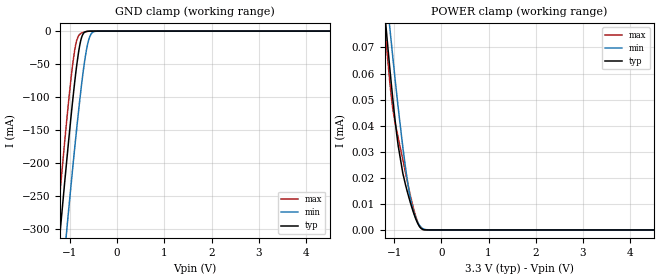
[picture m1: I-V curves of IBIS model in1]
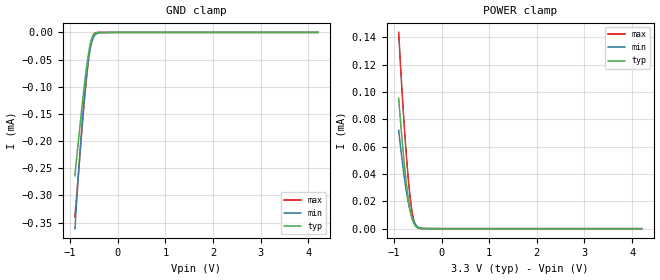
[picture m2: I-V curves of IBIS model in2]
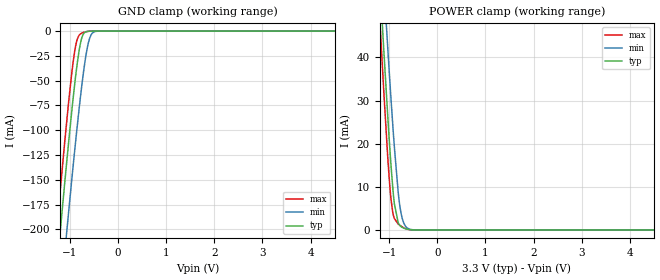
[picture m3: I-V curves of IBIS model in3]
|Texas Instruments Incorporated
|TPS53688 Dual-Channel (8+0, 7+1, 6+2, 5+3, 4+4 Phsases) D-CAP+ tm , Step Down
|Digital Multiphase Controller with VR13.HC and SVID
[IBIS Ver]   4.1
[File name]   tps53688.ibs
[Date]   25/04/2019
[File Rev]   1.0
[Source]
| Texas Instruments Incorporated.
| Analog-eLab Design Center, HPA
| 12500 TI Blvd
| Dallas, TX -75243
[Notes]   Revision History:
| Rev 1.0: 25/04/2019
| - Initial version of the model
| - Model generated from simulations in SPECTRE
| - C_comp although listed in numerical order of value are
|   obtained from varying PVT conditions. For PVT conditions for
|   each specific value refer the buffer description under
|   respective [Model]. IBIS model user is responsible for using
|   appropriate C_comp to simulate for Signal Integrity.
[Disclaimer]
| This model is designed as an aid for customers of Texas Instruments.
| TI and its licensors and suppliers make no warranties, either expressed
| or implied, with respect to this  model, including the warranties of
| merchantability or fitness for a particular purpose. The model is
| provided solely on an "as is" basis. The entire risk as to its quality
| and performance is with the customer.
| This model is subject to change without notice. Texas Instruments
| Incorporated is not responsible for updating this model.
[Copyright]
(C) Copyright 2019 Texas Instruments Incorporated.All rights reserved.
|  Component TPS53688RSB 40-Pin WQFN -RSB package
|  Part # TPS53688RSB
[Component]   TPS53688RSB
[Manufacturer]   TI
[Package]   |40 WQFN -RSB package
|   typ   min   max
R_pkg   0.05   0.04   0.06
L_pkg   1.0nH   0.8nH   1.2nH
C_pkg   0.2pF   0.16pF   0.24pF
[Pin] signal_name   model_name   R_pin   L_pin   C_pin
1   APWM8/BPWM1   out   NA   NA   NA
2   APWM7/BPWM2   out   NA   NA   NA
3   APWM6/BPWM3   out   NA   NA   NA
4   APWM5/BPWM4   out   NA   NA   NA
5   APWM4   out   NA   NA   NA
6   APWM3   out   NA   NA   NA
7   APWM2   out   NA   NA   NA
8   APWM1   out   NA   NA   NA
9   SMB_DIO   iood1   NA   NA   NA
10   SMB_CLK   iood1   NA   NA   NA
11   SMB_ALERTB   od1   NA   NA   NA
12   AVR_RDY   od2   NA   NA   NA
13   AVR_EN   in1   NA   NA   NA
14   VR_HOTB   od3   NA   NA   NA
15   PIN_ALT/PSYS_CRITB   od4   NA   NA   NA
16   BVR_RDY   od2   NA   NA   NA
17   SV_CLK   in2   NA   NA   NA
18   SV_DIO   iood2   NA   NA   NA
19   SV_ALERTB   iood2   NA   NA   NA
20   BVR_EN/VCCIO   in3   NA   NA   NA
21   AVSP   NC   NA   NA   NA
22   AVSN   NC   NA   NA   NA
23   ACSP1   NC   NA   NA   NA
24   ACSP2   NC   NA   NA   NA
25   ACSP3   NC   NA   NA   NA
26   ACSP4   NC   NA   NA   NA
27   ACSP5/BCSP4   NC   NA   NA   NA
28   ACSP6/BCSP3   NC   NA   NA   NA
29   ACSP7/BCSP2   NC   NA   NA   NA
30   ACSP8/BCSP1   NC   NA   NA   NA
31   BVSN   NC   NA   NA   NA
32   BVSP   NC   NA   NA   NA
33   VR_FAULTB   od5   NA   NA   NA
34   ADDR_CONFIG   NC   NA   NA   NA
35   BTSEN/TSEN   NC   NA   NA   NA
36   ATSEN/ISYS_IN   NC   NA   NA   NA
37   CSPIN   NC   NA   NA   NA
38   VIN_CSNIN   NC   NA   NA   NA
39   VCC   POWER   NA   NA   NA
40   VREF   NC   NA   NA   NA
| Models and submodels in the file (11): in1 (Input), in2 (Input), in3 (Input), iood1 (I/O_open_drain), iood2 (I/O_open_drain), od1 (Open_drain), od2 (Open_drain), od3 (Open_drain), od4 (Open_drain), od5 (Open_drain), out (3-state)
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|   in1 Model
[Model]   in1
Model_type   Input
Vinl = 0.725
Vinh = 0.775
|   typ   min   max
C_comp   1.478pF   1.451pF   1.505pF
[Voltage Range]   3.3   2.95   3.6
|Junction Temperature
[Temperature Range]   25   125   -40
[Power Clamp Reference]   3.3   2.95   3.6
[GND Clamp Reference]   0   0   0
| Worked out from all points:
|   GND clamp passes 1 mA (typ) near -0.67 V on its own axis
[GND Clamp]
|   Voltage   I(typ)   I(min)   I(max)
-3.3V     -2.068A    -2.144A    -2.033A
-1.28V    -362.5mA   -467.4mA   -301.6mA
-1.201V   -299.5mA   -405mA     -237.9mA
-1.102V   -222.5mA   -328.2mA   -161mA
-1.033V   -170.5mA   -275.6mA   -110.1mA
-943.8mV  -107.1mA   -209.7mA   -52.07mA
-874.5mV  -62.71mA   -160.3mA   -19.53mA
-795.3mV  -22.98mA   -107.2mA   -5.082mA
-735.9mV  -6.506mA   -71.08mA   -2.45mA
-597.3mV  -165.9uA   -12.28mA   -201.4uA
-468.6mV  -5.496uA   -501.9uA   -5.334uA
6.6V      0A         0A         0A
[POWER Clamp]
|   Voltage   I(typ)   I(min)   I(max)
-3.3V     563.7uA    525.3uA    632uA
-1.27V    98.59uA    111.2uA    95.86uA
-1.181V   80.02uA    94.34uA    75.26uA
-1.152V   74.01uA    88.81uA    68.81uA
-1.082V   60.46uA    76.12uA    55.17uA
-1.023V   49.58uA    65.54uA    45.96uA
-914.1mV  32.46uA    47.08uA    35.57uA
-815.1mV  21.76uA    31.8uA     26.95uA
-696.3mV  13.13uA    16.5uA     16.63uA
-547.8mV  4.581uA    4.947uA    5.62uA
-399.3mV  298.2nA    615.1nA    238.5nA
6.6V      0A         0A         0A
|   in2 Model
[Model]   in2
Model_type   Input
Vinl = 0.3
Vinh = 0.8
|   typ   min   max
C_comp   0.004pF   0.004pF   0.005pF
[Voltage Range]   3.3   2.95   3.6
|Junction Temperature
[Temperature Range]   25   125   -40
[Power Clamp Reference]   3.3   2.95   3.6
[GND Clamp Reference]   0   0   0
[GND Clamp]
|   Voltage   I(typ)   I(min)   I(max)
-900mV    -263.5uA   -361uA     -339.2uA
-838.8mV  -210.1uA   -278uA     -274.1uA
-762.3mV  -145.4uA   -183.1uA   -189.3uA
-716.4mV  -108.3uA   -133uA     -140.7uA
-660.3mV  -67.15uA   -81.67uA   -86.93uA
-609.3mV  -36.25uA   -46.32uA   -46.25uA
-558.3mV  -14.65uA   -22.38uA   -17.48uA
-532.8mV  -8.053uA   -14.45uA   -8.819uA
-507.3mV  -4.025uA   -8.873uA   -3.836uA
-451.2mV  -700.8nA   -2.661uA   -424.7nA
-12.6mV   0A         0A         0A
4.2V      0A         0A         0A
[POWER Clamp]
|   Voltage   I(typ)   I(min)   I(max)
-900mV    95.49uA    72.05uA    143.7uA
-843.9mV  71.19uA    54.65uA    109.1uA
-792.9mV  51.37uA    40.45uA    80.5uA
-741.9mV  34.23uA    28.12uA    55.13uA
-690.9mV  20.36uA    18.03uA    33.78uA
-645mV    11.18uA    11.1uA     18.84uA
-609.3mV  6.321uA    7.157uA    10.48uA
-568.5mV  2.935uA    4.053uA    4.526uA
-517.5mV  980.2nA    1.83uA     1.241uA
-395.1mV  49.66nA    218.8nA    26.95nA
-12.6mV   0A         0A         0A
4.2V      0A         0A         0A
|   in3 Model
[Model]   in3
Model_type   Input
Vinl = 0.3
Vinh = 0.8
|   typ   min   max
C_comp   1.658pF   1.628pF   1.689pF
[Voltage Range]   3.3   2.95   3.6
|Junction Temperature
[Temperature Range]   25   125   -40
[Power Clamp Reference]   3.3   2.95   3.6
[GND Clamp Reference]   0   0   0
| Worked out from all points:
|   GND clamp passes 1 mA (typ) near -0.68 V on its own axis
|   POWER clamp passes 1 mA (typ) near -0.78 V on its own axis
[GND Clamp]
|   Voltage   I(typ)   I(min)   I(max)
-3.3V     -1.398A    -1.448A    -1.375A
-1.28V    -242.8mA   -313mA     -202mA
-1.201V   -200.3mA   -270.9mA   -159mA
-1.102V   -148.6mA   -219.3mA   -107.3mA
-1.033V   -113.6mA   -183.9mA   -73.12mA
-943.8mV  -71.19mA   -139.8mA   -34.2mA
-884.4mV  -45.48mA   -111.4mA   -14.95mA
-795.3mV  -15.02mA   -71.26mA   -3.318mA
-735.9mV  -4.233mA   -47.12mA   -1.624mA
-617.1mV  -192.3uA   -11.49mA   -224.5uA
-468.6mV  -4.8uA     -332.7uA   -4.371uA
6.6V      0A         0A         0A
[POWER Clamp]
|   Voltage   I(typ)   I(min)   I(max)
-3.3V     505.9mA    511.8mA    523mA
-1.29V    76.52mA    91.81mA    67.94mA
-1.122V   43.33mA    59.06mA    33.77mA
-1.112V   41.45mA    57.18mA    31.82mA
-1.033V   26.71mA    42.52mA    17.15mA
-963.6mV  14.97mA    30.37mA    7.105mA
-894.3mV  6.118mA    19.32mA    2.661mA
-795.3mV  1.301mA    6.902mA    1.218mA
-745.8mV  709.2uA    3.408mA    828.2uA
-696.3mV  421.1uA    1.567mA    509.9uA
-448.8mV  5.18uA     16.56uA    2.962uA
6.6V      0A         0A         0A
